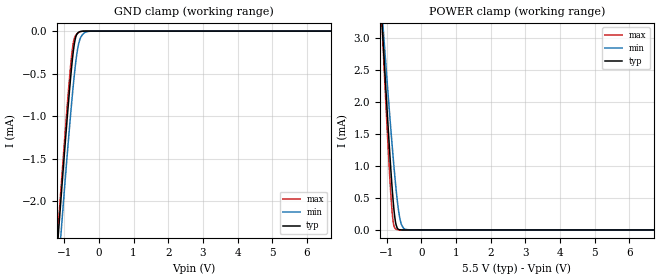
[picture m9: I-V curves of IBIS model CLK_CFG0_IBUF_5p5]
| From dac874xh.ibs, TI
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|   CLK_CFG0_IBUF_5p5 Model
[Model]   CLK_CFG0_IBUF_5p5
Model_type   Input
Vinl = 1.65
Vinh = 3.85
|   typ   min   max
C_comp   1.62855E-13  6.2518E-14   2.17306E-13
| Where nom  PVT is Nominal Process, 5.5V, 27C
|   Fast PVT is Strong Process,  5.501V, -40C
|   Slow PVT is Weak Process,   5.499V, 150C
[Model spec]
|subparameter
Vinl   1.65   1.6497   1.6503
Vinh   3.85   3.8493   3.8507
[Voltage Range]   5.5   5.499   5.501
[Temperature Range]   27   150   -40
[Power Clamp Reference]   5.5   5.499   5.501
[GND Clamp Reference]   0   0   0
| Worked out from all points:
|   GND clamp passes 1 mA (typ) near -0.91 V on its own axis
|   POWER clamp passes 1 mA (typ) near -0.89 V on its own axis
[GND Clamp]
|   Voltage   I(typ)   I(min)   I(max)
-5.5V     -27.53mA   -27.33mA   -27.99mA
-1.359V   -3.455mA   -3.822mA   -3.362mA
-1.177V   -2.442mA   -2.84mA    -2.331mA
-1.161V   -2.351mA   -2.751mA   -2.238mA
-1.127V   -2.17mA    -2.576mA   -2.053mA
-1.028V   -1.633mA   -2.054mA   -1.506mA
-880mV    -864.2uA   -1.3mA     -722.9uA
-781mV    -409uA     -832uA     -276.7uA
-682mV    -97.73uA   -425uA     -61.69uA
-550mV    -7.189uA   -102.1uA   -9.792uA
-220mV    0A         -175nA     0A
11V       0A         0A         0A
[POWER Clamp]
|   Voltage   I(typ)   I(min)   I(max)
-5.5V     48.9mA     43.04mA    56.37mA
-1.127V   3.188mA    3.353mA    3.146mA
-1.095V   2.874mA    3.109mA    2.773mA
-929.5mV  1.364mA    1.92mA     1.009mA
-847mV    695.3uA    1.358mA    313.7uA
-814mV    465.7uA    1.144mA    139.5uA
-764.5mV  197.5uA    840.9uA    30.44uA
-698.5mV  33.27uA    485uA      5.275uA
-632.5mV  3.608uA    220.1uA    915nA
-566.5mV  311.4nA    76.33uA    64.75nA
-302.5mV  0A         81.52nA    0A
11V       0A         0A         0A
